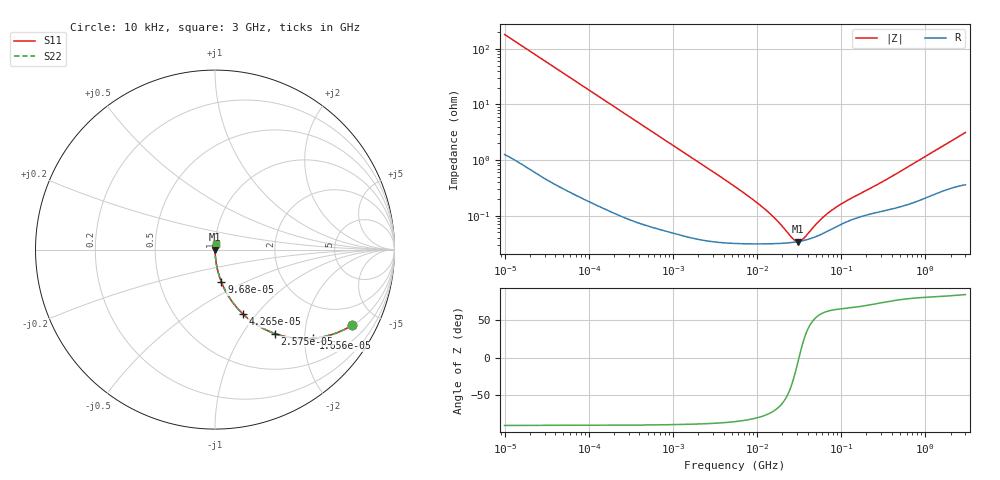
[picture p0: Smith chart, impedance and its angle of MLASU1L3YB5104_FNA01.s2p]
! MLASU1L3YB5104_FNA01  S-PARAMETER MODEL  ( Standard Model )
! Model Generated by TAIYO YUDEN Corporation (http://www.ty-top.com)
! Version 1.0
! TAIYO YUDEN Control No. 220601
! Copyright(c) 2014 TAIYO YUDEN CO.,LTD. All Rights Reserved.
! Product Description (link to TY-COMPAS)
! https://ds.yuden.co.jp/TYCOMPAS/or/detail?pn=MLASU1L3YB5104KFNA01&u=M
! Products Name : Multilayer Ceramic Capacitors
! Characteristics :
!  Capacitance : 0.1 [uF] , Rated Voltage : 50 [V] , TCC : X5R
!  Case Size : 1.0 x 0.5 / 0.039 x 0.02 [mm/inch] , Thickness : 0.3 / 0.012 [mm/inch]
!  (Conditions: Temperature = 25 [degC] , DC Bias Voltage = 0 [V])
! External Node Assignments :
!  1  o---| |---o  2
! GND o---------o GND
! Frequency Range : 10kHz  -  3GHz  [ 401 STEP ]
# MHZ S RI R 50
! Freq[MHz].  S11 Real  S11 Imag  S21 Real  S21 Imag  S12 Real  S12 Imag  S22 Real  S22 Imag
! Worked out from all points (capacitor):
!   401 points, 10 kHz to 3 GHz, reference 50 ohm
!   read as one part in series: C = 87.8 nF near 10.65 kHz
!   lowest |Z| = 34.4 mohm at 31.02 MHz (marker M1)
!   series resonance near 31.54 MHz, so ESL is about 290 pH
!   S11 on the Smith chart (normalised r, x): 10 kHz: 1.03, -3.62; 16.56 kHz: 1.02, -2.19; 25.75 kHz: 1.01, -1.41; 42.65 kHz: 1.01, -0.85; 96.8 kHz: 1.00, -0.38; 3 GHz: 1.01, +0.06
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0.01  0.7645 -0.4208  0.2355 0.4208  0.2355 0.4208  0.7645 -0.4208
0.012083  0.6908 -0.4586  0.3092 0.4586  0.3092 0.4586  0.6908 -0.4586
0.016561  0.5453 -0.4943  0.4547 0.4943  0.4547 0.4943  0.5453 -0.4943
0.02575  0.3339 -0.4679  0.6661 0.4679  0.6661 0.4679  0.3339 -0.4679
0.042645  0.1564 -0.3592  0.8436 0.3592  0.8436 0.3592  0.1564 -0.3592
0.058452  0.0908 -0.2831  0.9092 0.2831  0.9092 0.2831  0.0908 -0.2831
0.082683  0.0484 -0.2099  0.9516 0.2099  0.9516 0.2099  0.0484 -0.2099
0.096801  0.0361 -0.1818  0.9639 0.1818  0.9639 0.1818  0.0361 -0.1818
0.226771  0.00752 -0.0804  0.9925 0.0804  0.9925 0.0804  0.00752 -0.0804
0.683653  0.0013 -0.027  0.9987 0.027  0.9987 0.027  0.0013 -0.027
5.477226  0.000328 -0.00331  0.9997 0.00331  0.9997 0.00331  0.000328 -0.00331
12.83117  0.000313 -0.00122  0.9997 0.00122  0.9997 0.00122  0.000313 -0.00122
17.5871  0.000316 -0.000734  0.9997 0.000734  0.9997 0.000734  0.000316 -0.000734
26.49725  0.000331 -0.000208  0.9997 0.000208  0.9997 0.000208  0.000331 -0.000208
29.12589  0.000338 -9.44e-05  0.9997 9.44e-05  0.9997 9.44e-05  0.000338 -9.44e-05
31.02164  0.000343 -1.94e-05  0.9997 1.94e-05  0.9997 1.94e-05  0.000343 -1.94e-05
35.19136  0.000356 0.00013  0.9996 -0.00013  0.9996 -0.00013  0.000356 0.00013
45.28751  0.000397 0.000433  0.9996 -0.000433  0.9996 -0.000433  0.000397 0.000433
62.07353  0.000487 0.000827  0.9995 -0.000827  0.9995 -0.000827  0.000487 0.000827
87.80663  0.000637 0.00128  0.9994 -0.00128  0.9994 -0.00128  0.000637 0.00128
374.4521  0.00131 0.00461  0.9987 -0.00461  0.9987 -0.00461  0.00131 0.00461
3000  0.00455 0.0309  0.9954 -0.0309  0.9954 -0.0309  0.00455 0.0309
